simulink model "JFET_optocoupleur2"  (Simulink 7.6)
settings: Solver=ode15s  StartTime=0.0  StopTime=10  RelTol=1e-3
libraries: elec_lib x7, fl_lib x5, nesl_utility x3

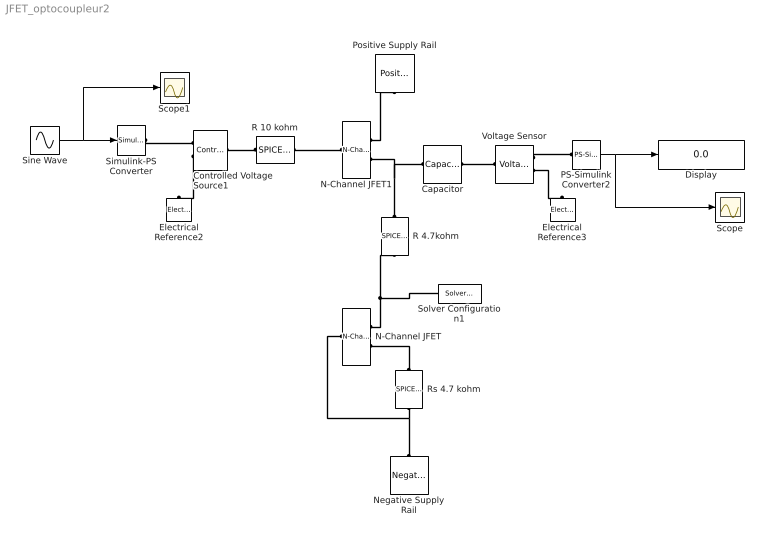
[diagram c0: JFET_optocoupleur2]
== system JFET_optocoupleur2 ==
  Capacitor : fl_lib/Electrical/Electrical Elements/Capacitor  DialogController=NetworkEngine.DynNeDlgSource  SystemSampleTime=-1  c=10e-6 F  v0=0 V  r=1e-6 Ohm  g=0 1/Ohm  i_Log=off  v_Log=off  vc_Log=off  LocalVarNames=|i|v|vc  LocalVarDescs=|i|v|Internal variable for voltage across capacitor term  LocalVarLogging=[0 0 0]
  Controlled Voltage Source1 : fl_lib/Electrical/Electrical Sources/Controlled Voltage Source  DialogController=NetworkEngine.DynNeDlgSource  SystemSampleTime=-1  i_Log=off  v_Log=off  LocalVarNames=|current|voltage|power  LocalVarDescs=|Current (A)|Voltage (V)|Power (W)  LocalVarLogging=[0 0 0]
  Display : Display
  Electrical Reference2 : fl_lib/Electrical/Electrical Elements/Electrical Reference  DialogController=NetworkEngine.DynNeDlgSource  SystemSampleTime=-1  i_Log=off  LocalVarNames=|i  LocalVarDescs=|i  LocalVarLogging=[]
  Electrical Reference3 : fl_lib/Electrical/Electrical Elements/Electrical Reference  DialogController=NetworkEngine.DynNeDlgSource  SystemSampleTime=-1  i_Log=off  LocalVarNames=|i  LocalVarDescs=|i  LocalVarLogging=[]
  N-Channel JFET : elec_lib/Semiconductor Devices/N-Channel JFET  DialogController=NetworkEngine.DynNeDlgSource  SystemSampleTime=-1  parameterization=1  Igss=-1 nA  Idss=17 mA  Idss_v="[  0 15 ] V"  ssig="[  3e+03 10 ] uS"  ssig_v="[  0 15 ] V"  Beta=1e-04 A/V^2  IS=1e-14 A  Tmeas=25 C  Vt0=-2 V  Lchannel=0 1/V  RS=0.1 Ohm  RD=0.1 Ohm  C_param=1  C_GS=3 pF  C_GD=1.5 pF  C_iss=4.5 pF  C_rss=1.5 pF  LocalVarLogging=[]
  N-Channel JFET1 : elec_lib/Semiconductor Devices/N-Channel JFET  DialogController=NetworkEngine.DynNeDlgSource  SystemSampleTime=-1  parameterization=1  Igss=-1 nA  Idss=17 mA  Idss_v="[  0 15 ] V"  ssig="[  3e+03 10 ] uS"  ssig_v="[  0 15 ] V"  Beta=1e-04 A/V^2  IS=1e-14 A  Tmeas=25 C  Vt0=-2 V  Lchannel=0 1/V  RS=0.1 Ohm  RD=0.1 Ohm  C_param=1  C_GS=3 pF  C_GD=1.5 pF  C_iss=4.5 pF  C_rss=1.5 pF  LocalVarLogging=[]
  Negative Supply Rail : elec_lib/Sources/Negative Supply Rail  DialogController=NetworkEngine.DynNeDlgSource  SystemSampleTime=-1  v0=-15 V  current_Log=off  voltage_Log=off  power_Log=off  LocalVarNames=|current|voltage|power  LocalVarDescs=|Current (A)|Voltage (V)|Power (W)  LocalVarLogging=[0 0 0]
  PS-Simulink Converter2 : nesl_utility/PS-Simulink Converter  DialogController=NetworkEngine.DynNeUtilDlgSource  SystemSampleTime=-1  PhysicalDomain=network_engine_domain  LeftPortType=input  RightPortType=output  SubClassName=ps_output  Unit=1  AffineConversion=off
  Positive Supply Rail : elec_lib/Sources/Positive Supply Rail  DialogController=NetworkEngine.DynNeDlgSource  SystemSampleTime=-1  v0=15 V  current_Log=off  voltage_Log=off  power_Log=off  LocalVarNames=|current|voltage|power  LocalVarDescs=|Current (A)|Voltage (V)|Power (W)  LocalVarLogging=[0 0 0]
  R 10 kohm : elec_lib/Additional Components/SPICE-Compatible Components/Passive Devices/SPICE Resistor  DialogController=NetworkEngine.DynNeDlgSource  SystemSampleTime=-1  SCALE=1  R_param=1  R=10 kOhm  RSH=0 Ohm  LENGTH=1e-06 m  WIDTH=1e-06 m  NARROW=0 m  T_param=1  TC1=0 1/K  TC2=0 1/K^2  TOFFSET=0 K  TFIXED=300.15 K  TMEAS=300.15 K  LocalVarLogging=[]
  R 4.7kohm : elec_lib/Additional Components/SPICE-Compatible Components/Passive Devices/SPICE Resistor  DialogController=NetworkEngine.DynNeDlgSource  SystemSampleTime=-1  SCALE=1  R_param=1  R=4.7 kOhm  RSH=0 Ohm  LENGTH=1e-06 m  WIDTH=1e-06 m  NARROW=0 m  T_param=1  TC1=0 1/K  TC2=0 1/K^2  TOFFSET=0 K  TFIXED=300.15 K  TMEAS=300.15 K  LocalVarLogging=[]
  Rs 4.7 kohm : elec_lib/Additional Components/SPICE-Compatible Components/Passive Devices/SPICE Resistor  DialogController=NetworkEngine.DynNeDlgSource  SystemSampleTime=-1  SCALE=1  R_param=1  R=4.7 kOhm  RSH=0 Ohm  LENGTH=1e-06 m  WIDTH=1e-06 m  NARROW=0 m  T_param=1  TC1=0 1/K  TC2=0 1/K^2  TOFFSET=0 K  TFIXED=300.15 K  TMEAS=300.15 K  LocalVarLogging=[]
  Scope : Scope
  Scope1 : Scope
  Simulink-PS Converter : nesl_utility/Simulink-PS Converter  DialogController=NetworkEngine.DynNeUtilDlgSource  SystemSampleTime=-1  PhysicalDomain=network_engine_domain  LeftPortType=input  RightPortType=output  SubClassName=ps_input  Unit=1  AffineConversion=off  InputFilterTimeConstant=.001  UdotUserProvided=0
  Sine Wave : Sin  SampleTime=0
  Solver Configuration1 : nesl_utility/Solver Configuration  DialogController=NetworkEngine.DynNeUtilDlgSource  SystemSampleTime=-1  PhysicalDomain=network_engine_domain  LeftPortType=input  RightPortType=generic  SubClassName=solver  Accelerate=off  Profile=off  ResidualTolerance=1e-9  MaxNonlinIter=12  MaxModeIter=2  DoFixedCost=off  UseLocalSampling=off  DoDC=off  LinearAlgebra=Sparse  LocalSolverSampleTime=.001  LocalSolverChoice=NE_BACKWARD_EULER_ADVANCER  UseLocalSolver=off
  Voltage Sensor : fl_lib/Electrical/Electrical Sensors/Voltage Sensor  DialogController=NetworkEngine.DynNeDlgSource  SystemSampleTime=-1  i1_Log=off  v1_Log=off  LocalVarNames=|i1|v1  LocalVarDescs=|i1|v1  LocalVarLogging=[0 0]
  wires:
  PS-Simulink Converter2/1 -> Display/1, Scope/1
  Sine Wave/1 -> Simulink-PS Converter/1, Scope1/1
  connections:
  Rs 4.7 kohm/RConn1 -- Negative Supply Rail/LConn1 -- N-Channel JFET/LConn1
  Rs 4.7 kohm/LConn1 -- N-Channel JFET/RConn2
  Voltage Sensor/RConn2 -- Electrical Reference3/LConn1
  Voltage Sensor/RConn1 -- PS-Simulink Converter2/LConn1
  N-Channel JFET1/RConn1 -- Positive Supply Rail/RConn1
  R 4.7kohm/LConn1 -- N-Channel JFET1/RConn2 -- Capacitor/LConn1
  N-Channel JFET/RConn1 -- R 4.7kohm/RConn1 -- Solver Configuration1/RConn1
  R 10 kohm/RConn1 -- N-Channel JFET1/LConn1
  Controlled Voltage Source1/LConn1 -- R 10 kohm/LConn1
  Simulink-PS Converter/RConn1 -- Controlled Voltage Source1/RConn1
  Controlled Voltage Source1/RConn2 -- Electrical Reference2/LConn1
  Capacitor/RConn1 -- Voltage Sensor/LConn1
